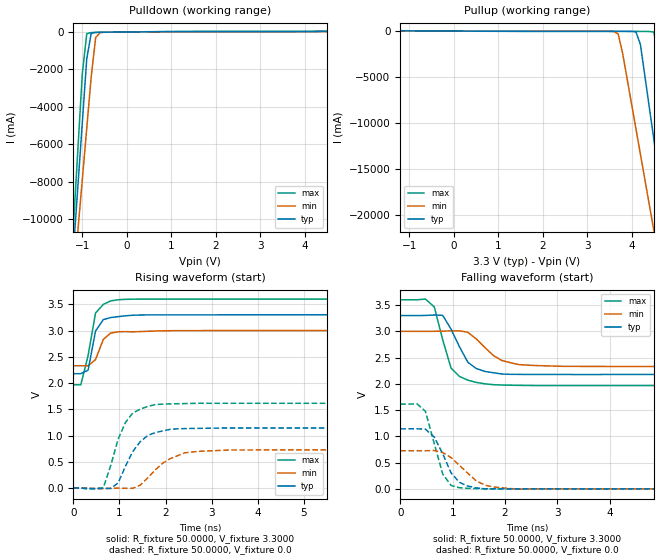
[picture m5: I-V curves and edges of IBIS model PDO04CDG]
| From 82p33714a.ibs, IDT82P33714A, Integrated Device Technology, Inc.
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|   Model PDO04CDG
[Model]  PDO04CDG
Model_type Output
Polarity   Non-Inverting
Vmeas =  1.6500V
Cref =   50.0000pF
Rref =   1.0000M
Vref =   0.0V
C_comp   70.2000fF   57.9000fF   75.6000fF
[Temperature Range]   25.0000   0.1250k   -40.0000
[Voltage Range]   3.3000V   3.0000V   3.6000V
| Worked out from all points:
|   slope of the pulldown table from 0 to 0.495 V, typ, clamps not added: 46.8 ohm
|   slope of the pullup table from 0 to 0.495 V, typ, clamps not added: 51.6 ohm
|   rising waveform, R_fixture 50.0000, V_fixture 3.3000: 20-80 % time 192ps typ, 207ps min, 215ps max; typ from 2.18 V to 3.3 V
|   rising waveform, R_fixture 50.0000, V_fixture 0.0: 20-80 % time 459ps typ, 606ps min, 397ps max; typ from 0 V to 1.14 V
|   falling waveform, R_fixture 50.0000, V_fixture 3.3000: 20-80 % time 352ps typ, 467ps min, 277ps max; typ from 3.3 V to 2.18 V
|   falling waveform, R_fixture 50.0000, V_fixture 0.0: 20-80 % time 350ps typ, 480ps min, 267ps max; typ from 1.14 V to 0 V
[Pulldown]
|Voltage   I(typ)   I(min)   I(max)
-3.3V     -83.46A    -71.04A    -95.7A
-1.2V     -11.7A     -13.4A     -10.38A
-1.1V     -8.282A    -10.65A    -6.315A
-1V       -4.861A    -7.903A    -2.249A
-900mV    -1.44A     -5.154A    -86.78mA
-800mV    -73.23mA   -2.406A    -31.89mA
-700mV    -19.25mA   -307.3mA   -24.01mA
-600mV    -14.45mA   -31.58mA   -18.56mA
6.6V      61.77mA    24.65mA    92.18mA
[Pullup]
|Voltage   I(typ)   I(min)   I(max)
-3.3V     36.31mA    5.38mA     78.53mA
3.6V      -24.07mA   -38.01mA   -34.81mA
3.7V      -24.12mA   -314.9mA   -34.87mA
3.8V      -24.19mA   -2.415A    -34.92mA
4.1V      -81.37mA   -10.66A    -35.14mA
4.2V      -1.453A    -13.41A    -35.93mA
4.5V      -11.72A    -21.65A    -99.97mA
4.6V      -15.14A    -24.4A     -2.27A
4.8V      -21.98A    -29.9A     -10.4A
5V        -28.82A    -35.39A    -18.54A
5.1V      -32.24A    -38.14A    -22.6A
6.6V      -83.49A    -79.28A    -83.56A
[Ramp]
| variable   typ   min   max
dV/dt_r  0.6858/0.4559n   0.4358/0.6023n   0.9684/0.3971n
dV/dt_f  0.6732/0.3519n   0.4020/0.4573n   0.9798/0.2768n
R_load = 50.0000
[Rising Waveform]
R_fixture= 50.0000
V_fixture= 3.3000
V_fixture_min= 3.0000
V_fixture_max= 3.6000
L_fixture= 0.0H
C_fixture= 0.0F
|time   V(typ)   V(min)   V(max)
0s        2.178V     2.33V      1.967V
160ps     2.178V     2.33V      1.966V
320ps     2.246V     2.328V     2.53V
480ps     2.991V     2.447V     3.333V
650ps     3.209V     2.833V     3.499V
810ps     3.248V     2.952V     3.565V
970ps     3.265V     2.977V     3.587V
1.29ns    3.292V     2.976V     3.598V
1.78ns    3.299V     2.992V     3.599V
16ns      3.3V       3V         3.6V
[Rising Waveform]
R_fixture= 50.0000
V_fixture= 0.0
V_fixture_min= 0.0
V_fixture_max= 0.0
L_fixture= 0.0H
C_fixture= 0.0F
|time   V(typ)   V(min)   V(max)
0s        5.065uV    5.682uV    4.766uV
650ps     -6.501mV   -12.91mV   6.703mV
970ps     96.75mV    -2.898mV   929.3mV
1.13ns    414.5mV    -5.596mV   1.25V
1.29ns    697.9mV    -5.314mV   1.431V
1.45ns    881.8mV    54.83mV    1.502V
1.78ns    1.056V     348.1mV    1.59V
2.42ns    1.132V     670.8mV    1.609V
3.39ns    1.144V     723.5mV    1.614V
16ns      1.143V     726.3mV    1.614V
[Falling Waveform]
R_fixture= 50.0000
V_fixture= 3.3000
V_fixture_min= 3.0000
V_fixture_max= 3.6000
L_fixture= 0.0H
C_fixture= 0.0F
|time   V(typ)   V(min)   V(max)
0s        3.3V       3V         3.6V
480ps     3.302V     2.999V     3.614V
650ps     3.311V     3V         3.464V
810ps     3.304V     3.004V     2.838V
970ps     3.04V      3.008V     2.299V
1.29ns    2.41V      2.982V     2.07V
1.62ns    2.235V     2.687V     1.999V
2.1ns     2.181V     2.403V     1.974V
3.07ns    2.178V     2.334V     1.967V
16ns      2.178V     2.33V      1.967V
[Falling Waveform]
R_fixture= 50.0000
V_fixture= 0.0
V_fixture_min= 0.0
V_fixture_max= 0.0
L_fixture= 0.0H
C_fixture= 0.0F
|time   V(typ)   V(min)   V(max)
0s        1.143V     726.3mV    1.614V
320ps     1.144V     726.1mV    1.618V
480ps     1.136V     726.4mV    1.478V
650ps     984.6mV    730.5mV    859.8mV
810ps     670.8mV    692.4mV    282.1mV
970ps     302.4mV    595mV      65.46mV
1.13ns    123.9mV    448mV      21.86mV
1.62ns    1.071mV    69.29mV    1.177mV
2.26ns    384.9uV    -5.533mV   -21.92uV
16ns      -978.3nV   27.26uV    -5.154uV
